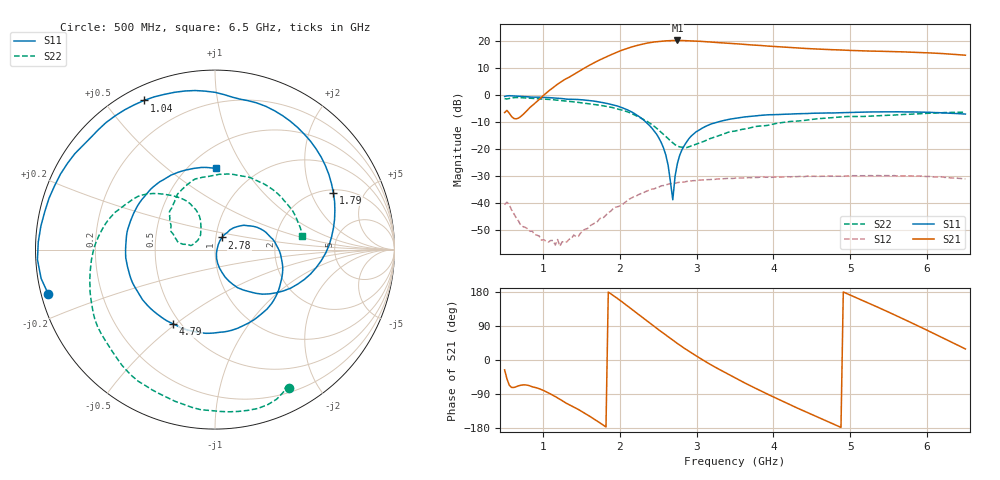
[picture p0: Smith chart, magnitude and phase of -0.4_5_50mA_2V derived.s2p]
!Agilent Technologies,E8363B,MY43030569,A.06.01.05
!Agilent E8363B: A.06.01.05
!Date: Tuesday, July 21, 2009 12:50:26
!Correction: S11(Full 2 Port(1,2)) S21(Full 2 Port(1,2)) S12(Full 2 Port(1,2)) S22(Full 2 Port(1,2))
!S2P File: Measurements: S11, S21, S12, S22:
# Hz S  dB  R 50
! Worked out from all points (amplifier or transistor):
!   201 points, 500 MHz to 6.5 GHz, reference 50 ohm
!   highest |S21| = 20.4 dB at 2.75 GHz (marker M1)
!   |S21| within 3 dB of that: 2.089 GHz to 4.45 GHz (2.361 GHz wide, 72.2 % of centre)
!   unconditionally stable (mu >= 1): start of sweep to end of sweep
!   at 1.49 GHz: K = 8.95, MAG = 17.6 dB, |S12| = -51.0 dB
!   at 3.5 GHz: K = 1.66, MAG = 20.1 dB, |S12| = -30.6 dB
!   at 6.5 GHz: K = 1.78, MAG = 17.8 dB, |S12| = -30.9 dB
!   S11 on the Smith chart (normalised r, x): 500 MHz: 0.02, -0.13; 1.04 GHz: 0.06, +0.63; 1.79 GHz: 2.14, +2.93; 2.78 GHz: 1.07, +0.15; 4.79 GHz: 0.46, -0.49; 6.5 GHz: 0.67, +0.76
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5e8  -0.34 -165.0  -6.33 -26.0  -40.44 86.8  -1.16 -61.9
1.04e9  -0.72 115.5  0.85 -83.7  -54.05 -79.7  -1.40 -117.1
1.52e9  -1.63 59.6  9.82 -137.5  -50.01 -171.6  -2.80 -164.0
1.79e9  -2.71 25.7  13.85 -172.6  -45.18 150.7  -3.86 170.6
2e9  -4.19 -1.8  16.46 157.9  -40.93 120.5  -5.23 151.1
2.15e9  -6.02 -22.6  17.94 135.0  -37.99 99.5  -6.64 137.8
2.36e9  -10.38 -50.8  19.43 102.4  -35.30 69.9  -9.69 121.8
2.51e9  -15.80 -69.9  20.02 79.2  -33.89 47.9  -12.91 115.1
2.69e9  -38.62 7.8  20.36 52.4  -32.58 23.6  -17.55 126.4
2.75e9  -25.15 61.0  20.38 43.7  -32.28 16.5  -18.76 134.1
2.78e9  -22.14 60.4  20.38 39.4  -32.13 12.1  -19.03 138.0
2.93e9  -15.03 46.1  20.23 19.1  -31.62 -5.7  -18.68 159.6
3.11e9  -11.53 27.9  19.95 -3.4  -31.20 -25.4  -16.82 169.9
3.5e9  -8.47 -9.3  19.17 -47.2  -30.62 -63.9  -13.17 166.0
3.74e9  -7.62 -30.3  18.69 -71.9  -30.29 -84.3  -11.68 158.3
3.95e9  -7.13 -48.6  18.26 -92.7  -30.23 -103.7  -10.89 150.0
4.52e9  -6.57 -96.4  17.27 -145.6  -29.91 -150.2  -8.80 126.3
4.79e9  -6.47 -119.4  16.95 -169.7  -29.89 -172.2  -8.16 114.4
5.18e9  -6.17 -153.3  16.53 155.5  -29.72 156.0  -7.76 94.9
5.51e9  -6.06 177.5  16.29 125.4  -29.69 128.9  -7.30 76.2
5.96e9  -6.17 137.0  15.87 82.6  -29.92 89.8  -6.66 46.0
6.5e9  -6.88 89.1  14.92 29.1  -30.88 41.8  -6.22 8.9
